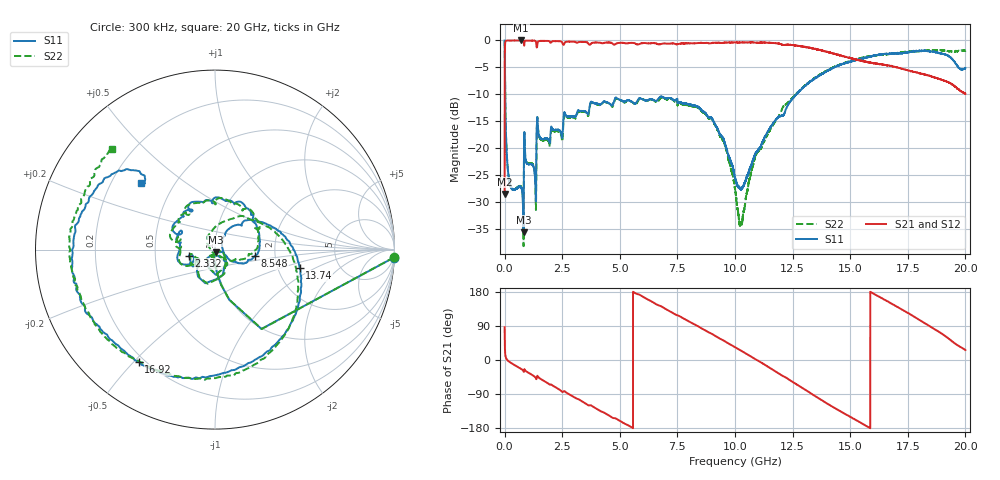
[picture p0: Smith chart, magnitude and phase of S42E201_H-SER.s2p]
! Created Wed Nov 25 22:05:56 2020
# khz S ma R 50
! 2 Port Network Data from SP1.SP block
! freq  magS11  angS11  magS21  angS21  magS12  angS12  magS22  angS22
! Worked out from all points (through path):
!   20001 points, 300 kHz to 20 GHz, reference 50 ohm
!   highest |S21| = -0.01 dB at 725.3 MHz (marker M1); lowest = -28.5 dB at 300 kHz (marker M2)
!   group delay of S21, straight-line fit = 96.1 ps
!   lowest |S11| = -35.5 dB at 820.3 MHz (marker M3), VSWR 1.03, Z = 50.5 - j1.59 ohm
!   |S11| at or under -10 dB: 23.86 MHz to 12.66 GHz (12.64 GHz wide, 199 % of centre)
!   |S22| runs from -38.1 to 0.0 dB; largest |S21 - S12| = 0.018
!   S11 on the Smith chart (normalised r, x): 300 kHz: 3, -45; 2.332 GHz: 0.75, -0.05; 8.548 GHz: 1.56, -0.12; 13.74 GHz: 2.65, -0.71; 16.92 GHz: 0.18, -0.52; 20 GHz: 0.32, +0.35
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300  0.9971 -2.6  0.03774 86.5  0.03778 87.3  0.9974 -2.5
102300  0.08244 -89.7  0.995 1.0  0.9961 1.0  0.08292 -89.4
201300  0.04965 -96.5  0.997 -4.5  0.9969 -4.4  0.05037 -96.5
725300  0.04309 -113.9  0.9986 -23.9  0.9975 -23.9  0.04357 -116.0
820300  0.01671 -70.6  0.9881 -29.3  0.9882 -29.2  0.01326 -82.7
1278300  0.06457 -132.0  0.9942 -42.9  0.9951 -42.9  0.06555 -133.7
1482300  0.133 -136.6  0.9832 -46.3  0.9835 -46.3  0.1357 -133.3
2332300  0.1484 -166.4  0.9838 -76.4  0.9837 -76.4  0.1447 -167.2
3334300  0.222 157.3  0.9686 -108.0  0.9669 -108.0  0.2186 166.3
5110300  0.2756 105.4  0.9503 -164.5  0.9491 -164.5  0.2737 107.8
6667300  0.2868 66.4  0.9215 144.6  0.9199 144.6  0.2738 55.1
8548300  0.2244 -9.1  0.9483 83.5  0.9459 83.6  0.2214 -1.2
1.00003e7  0.05379 -22.7  0.9581 33.8  0.9585 33.9  0.04251 -69.4
1.02743e7  0.04185 16.4  0.9575 24.2  0.9579 24.2  0.02027 -143.3
1.14933e7  0.1507 54.5  0.9495 -20.1  0.9485 -20.1  0.1441 81.2
1.33343e7  0.4228 3.3  0.8443 -89.7  0.848 -89.5  0.428 -4.2
1.37363e7  0.4826 -12.2  0.8089 -105.1  0.8148 -104.8  0.4877 -19.5
1.51603e7  0.6489 -67.5  0.6688 -155.3  0.6749 -155.9  0.6611 -64.7
1.66673e7  0.7494 -115.9  0.5876 153.5  0.5729 153.5  0.746 -116.8
1.69193e7  0.7568 -124.1  0.57 144.6  0.5556 144.9  0.7546 -125.9
1.83123e7  0.797 -175.8  0.4774 94.3  0.4799 95.2  0.8027 -171.1
2e7  0.5555 138.2  0.3203 26.4  0.3233 27.3  0.8011 135.4
